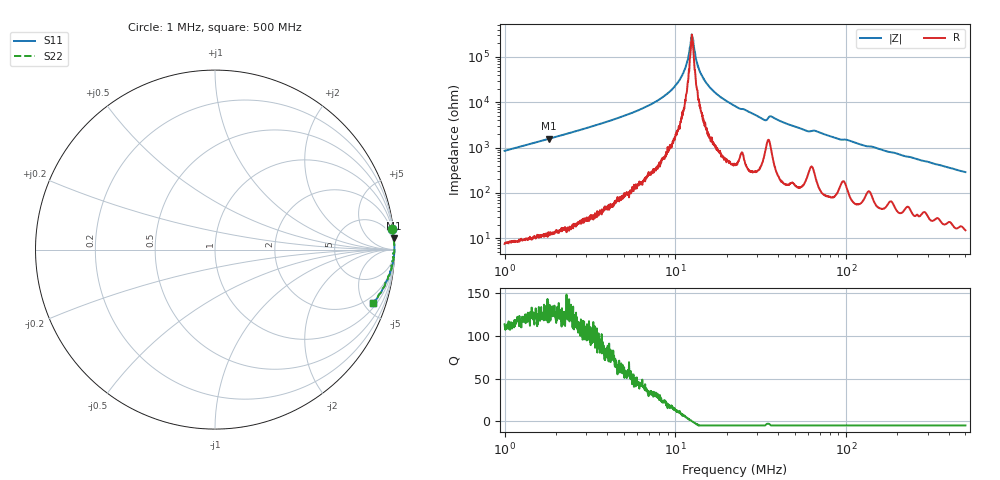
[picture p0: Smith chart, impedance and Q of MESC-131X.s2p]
!s-Parameter Generated by FASTRON Sdn. Bhd.
!FASTRON P/N : MESC-131X
!Keysight Technologies,E4991B,MY54100416,A.01.15
!Date: Fri Mar 27 09:49:21 2026
!Version  : Rev00 Fri Mar 27 09:49:21 2026
!Data & Calibration Information:
!PortZ  Port1:50+j0  Port2:50+j0
!When reading, reference impedance value at option line is always used.
!Remarks : This data is being provided solely for informational purposes.
!Freq	S11	S21	S12	S22
# Hz S dB R 50
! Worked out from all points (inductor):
!   1601 points, 1 MHz to 500 MHz, reference 50 ohm
!   read as one part in series: L = 134 uH near 1.032 MHz
!   highest Q = 133 at 1.819 MHz (marker M1), where L = 137 uH
!   self-resonance near 12.49 MHz
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1000000  -0.07 6.7  -18.64 -82.8  -18.64 -82.8  -0.07 6.7
1818762  -0.02 3.6  -23.92 -85.9  -23.92 -85.9  -0.02 3.6
2820919  -0.01 2.3  -27.97 -87.2  -27.97 -87.2  -0.01 2.3
5523530  -0.00 1.0  -35.18 -87.9  -35.18 -87.9  -0.00 1.0
7957584  -0.00 0.5  -41.03 -87.4  -41.03 -87.4  -0.00 0.5
9477412  -0.00 0.3  -45.36 -86.6  -45.36 -86.6  -0.00 0.3
1.069011e7  -0.00 0.2  -50.40 -83.6  -50.40 -83.6  -0.00 0.2
1.150887e7  -0.00 0.1  -55.67 -78.1  -55.67 -78.1  -0.00 0.1
1.229445e7  -0.00 0.0  -66.16 -45.2  -66.16 -45.2  -0.00 0.0
1.253555e7  -0.00 -0.0  -69.37 4.3  -69.37 4.3  -0.00 -0.0
1.278138e7  -0.00 -0.0  -65.64 50.2  -65.64 50.2  -0.00 -0.0
1.328759e7  -0.00 -0.1  -58.21 73.5  -58.21 73.5  -0.00 -0.1
1.370696e7  -0.00 -0.1  -55.07 77.9  -55.07 77.9  -0.00 -0.1
1.504616e7  -0.00 -0.2  -48.98 84.2  -48.98 84.2  -0.00 -0.2
1.757519e7  -0.00 -0.4  -43.52 85.8  -43.52 85.8  -0.00 -0.4
2.236068e7  -0.01 -0.7  -38.36 86.4  -38.36 86.4  -0.01 -0.7
3.310225e7  -0.04 -1.4  -32.30 79.7  -32.30 79.7  -0.04 -1.4
3.661978e7  -0.03 -1.2  -33.73 79.4  -33.73 79.4  -0.03 -1.2
5.79115e7  -0.04 -2.4  -27.59 83.3  -27.59 83.3  -0.04 -2.4
6.307767e7  -0.07 -2.4  -27.47 78.3  -27.47 78.3  -0.07 -2.4
1.77937e8  -0.15 -7.0  -18.24 78.7  -18.24 78.7  -0.15 -7.0
5e8  -0.63 -18.8  -9.81 68.2  -9.81 68.2  -0.63 -18.8
